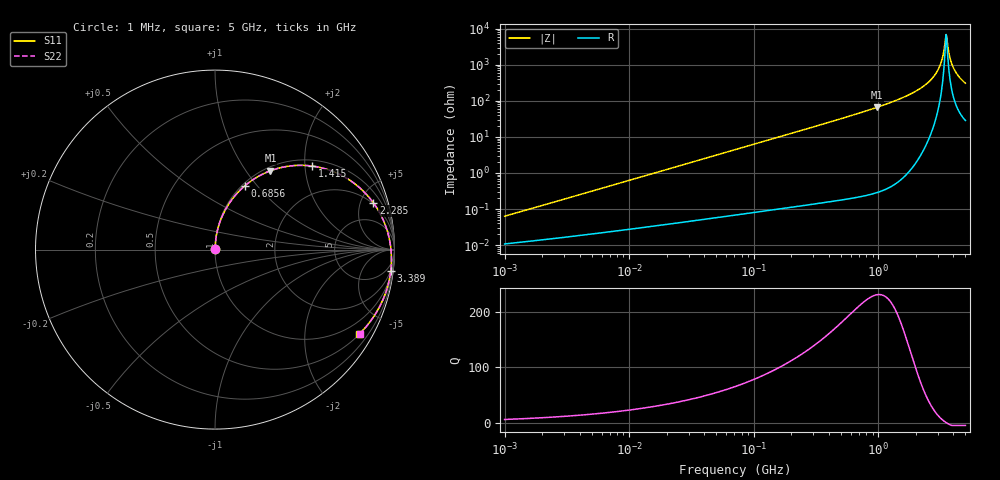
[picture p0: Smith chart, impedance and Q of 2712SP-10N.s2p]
# MHz  S  MA  R  50
!Freq  MagS11  AngS11  MagS21  AngS21  MagS12  AngS12  MagS22  AngS22
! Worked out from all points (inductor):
!   801 points, 1 MHz to 5 GHz, reference 50 ohm
!   read as one part in series: L = 9.92 nH near 1.044 MHz
!   highest Q = 231 at 974.4 MHz (marker M1), where L = 10.8 nH
!   self-resonance near 3.499 GHz
!   S11 on the Smith chart (normalised r, x): 1 MHz: 1.00, +0.00; 685.6 MHz: 1.03, +0.87; 1.415 GHz: 1.15, +2.18; 2.285 GHz: 1.88, +6.38; 3.389 GHz: 2, -16; 5 GHz: 0.51, -3.63
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1  0.0006118 79.8  0.9999 -0.0  0.9999 -0.0  0.0006118 79.8
4.168304  0.002517 85.6  0.9998 -0.2  0.9998 -0.2  0.002517 85.6
17.19065  0.01036 87.4  0.9996 -0.6  0.9996 -0.6  0.01035 87.4
70.89654  0.04266 86.5  0.9984 -2.6  0.9984 -2.6  0.04265 86.5
295.5183  0.1763 78.7  0.983 -10.9  0.983 -10.9  0.1763 78.7
685.6191  0.3945 64.8  0.917 -24.9  0.917 -24.9  0.3944 64.8
974.4498  0.5371 54.9  0.8412 -34.9  0.8412 -34.9  0.5369 54.9
1218.757  0.6417 46.8  0.764 -42.9  0.764 -42.9  0.6415 46.8
1414.781  0.7143 40.7  0.6962 -49.0  0.6962 -49.0  0.7141 40.7
1807.591  0.8295 29.1  0.5522 -60.5  0.5522 -60.5  0.8292 29.1
2284.991  0.9201 16.4  0.3768 -72.6  0.3768 -72.6  0.9199 16.4
2652.506  0.9601 7.8  0.2501 -80.3  0.2501 -80.3  0.9599 7.8
2982.281  0.979 0.8  0.146 -85.1  0.146 -85.1  0.9789 0.8
3213.176  0.9849 -3.7  0.07937 -85.0  0.07937 -85.0  0.9849 -3.7
3388.967  0.9862 -6.9  0.03339 -73.6  0.03339 -73.6  0.9863 -6.9
3461.947  0.9861 -8.2  0.01803 -48.6  0.01803 -48.6  0.9862 -8.2
3574.375  0.9851 -10.2  0.02212 38.6  0.02212 38.6  0.9853 -10.2
3651.348  0.9841 -11.4  0.03848 55.3  0.03848 55.3  0.9842 -11.4
3810.303  0.9808 -14.0  0.07419 63.2  0.07419 63.2  0.9811 -14.0
4018.762  0.9748 -17.3  0.119 64.0  0.119 64.0  0.9752 -17.3
4423.147  0.9591 -23.0  0.1966 60.8  0.1966 60.8  0.9597 -23.0
5000  0.9317 -30.3  0.2875 54.6  0.2875 54.6  0.9328 -30.3
